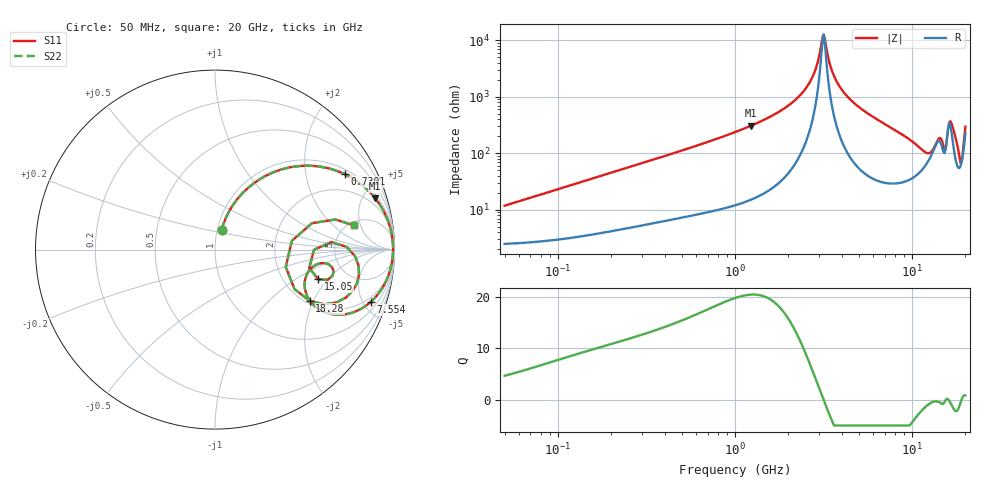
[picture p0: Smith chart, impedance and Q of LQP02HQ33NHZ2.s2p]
!Murata Part Number: LQP02HQ33NHZ2
!These Parameters are Measured in Series Mode Connection
!  o--[Z]--o
!Port1  Port2
!  o-------o
!Freq. Start=50[MHz] Stop=20[GHz], 401[Steps]
# Hz S RI R 50
!Freq.(Hz) S11(Real) S11(Imag) S21(Real) S21(Imag) S12(Real) S12(Imag) S22(Real) S22(Imag)
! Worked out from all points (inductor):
!   401 points, 50 MHz to 20 GHz, reference 50 ohm
!   read as one part in series: L = 36.6 nH near 51.52 MHz
!   highest Q = 20.4 at 1.233 GHz (marker M1), where L = 39.7 nH
!   self-resonance near 3.122 GHz
!   S11 on the Smith chart (normalised r, x): 50 MHz: 1.05, +0.23; 730.1 MHz: 1.19, +3.31; 7.554 GHz: 1.58, -5.72; 15.05 GHz: 3.09, -1.59; 18.28 GHz: 2.10, -1.88; 20 GHz: 5.49, +3.85
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5e7  0.0364 0.1085  0.9636 -0.1085  0.9636 -0.1085  0.0364 0.1085
1.364002e8  0.1127 0.2662  0.8873 -0.2662  0.8873 -0.2662  0.1127 0.2662
3.721004e8  0.4137 0.4574  0.5863 -0.4574  0.5863 -0.4574  0.4137 0.4574
7.30116e8  0.7219 0.4209  0.2781 -0.4209  0.2781 -0.4209  0.7219 0.4209
1e9  0.8363 0.3456  0.1637 -0.3456  0.1637 -0.3456  0.8363 0.3456
1.23331e9  0.8935 0.285  0.1065 -0.285  0.1065 -0.285  0.8935 0.285
2.05233e9  0.9739 0.1298  0.0261 -0.1298  0.0261 -0.1298  0.9739 0.1298
2.728004e9  0.9903 0.0444  0.0097 -0.0444  0.0097 -0.0444  0.9903 0.0444
3.168813e9  0.9922 -0.000561  0.00781 0.000561  0.00781 0.000561  0.9922 -0.000561
3.572216e9  0.9904 -0.0369  0.00964 0.0369  0.00964 0.0369  0.9904 -0.0369
4.087748e9  0.9844 -0.0787  0.0156 0.0787  0.0156 0.0787  0.9844 -0.0787
7.442007e9  0.8747 -0.2851  0.1253 0.2851  0.1253 0.2851  0.8747 -0.2851
7.554318e9  0.8688 -0.2906  0.1312 0.2906  0.1312 0.2906  0.8688 -0.2906
1.019291e10  0.6686 -0.3625  0.3314 0.3625  0.3314 0.3625  0.6686 -0.3625
1.201863e10  0.5064 -0.2406  0.4936 0.2406  0.4936 0.2406  0.5064 -0.2406
1.334722e10  0.5631 -0.0838  0.4369 0.0838  0.4369 0.0838  0.5631 -0.0838
1.504638e10  0.575 -0.1651  0.425 0.1651  0.425 0.1651  0.575 -0.1651
1.573793e10  0.648 0.0418  0.352 -0.0418  0.352 -0.0418  0.648 0.0418
1.646126e10  0.8003 -0.0905  0.1997 0.0905  0.1997 0.0905  0.8003 -0.0905
1.828096e10  0.5278 -0.2864  0.4722 0.2864  0.4722 0.2864  0.5278 -0.2864
1.912117e10  0.4283 0.0489  0.5717 -0.0489  0.5717 -0.0489  0.4283 0.0489
2e10  0.7721 0.1354  0.2279 -0.1354  0.2279 -0.1354  0.7721 0.1354
